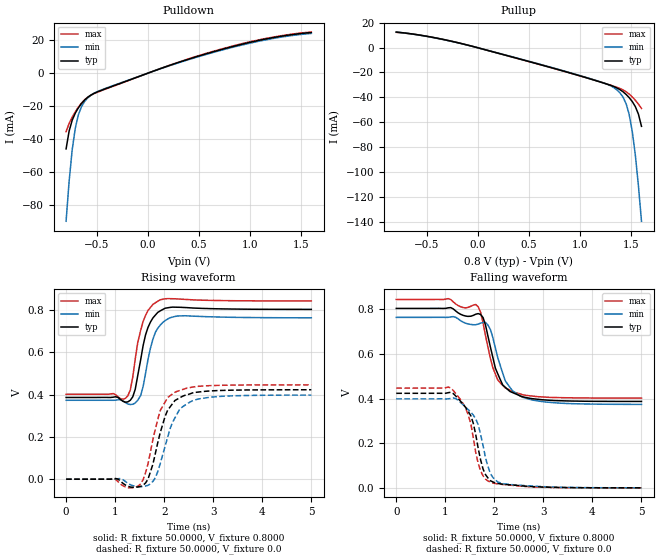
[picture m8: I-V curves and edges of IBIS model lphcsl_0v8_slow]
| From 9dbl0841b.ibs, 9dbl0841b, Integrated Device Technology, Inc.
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|   Model lphcsl_0v8_slow
[Model]  lphcsl_0v8_slow
Model_type Output
Polarity   Non-Inverting
Vmeas =  0.4000V
Cref =   2.0000pF
Rref =   0.0
Vref =   0.4000V
C_comp   1.1000pF   1.0000pF   1.2000pF
[Temperature Range]   27.0000   70.0000   0.0
[Voltage Range]   0.8000V   0.7600V   0.8400V
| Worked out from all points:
|   slope of the pulldown table from 0 to 0.12 V, typ, clamps not added: 44.4 ohm
|   slope of the pullup table from 0 to 0.12 V, typ, clamps not added: 45.4 ohm
|   rising waveform, R_fixture 50.0000, V_fixture 0.8000: 20-80 % time 229ps typ, 225ps min, 222ps max; typ from 0.387 V to 0.804 V
|   rising waveform, R_fixture 50.0000, V_fixture 0.0: 20-80 % time 326ps typ, 359ps min, 314ps max; typ from 0 V to 0.424 V
|   falling waveform, R_fixture 50.0000, V_fixture 0.8000: 20-80 % time 322ps typ, 361ps min, 304ps max; typ from 0.804 V to 0.387 V
|   falling waveform, R_fixture 50.0000, V_fixture 0.0: 20-80 % time 292ps typ, 304ps min, 288ps max; typ from 0.424 V to 0 V
[Pulldown]
|Voltage   I(typ)   I(min)   I(max)
-800mV    -45.83mA   -89.64mA   -35.38mA
-770mV    -34.96mA   -65.18mA   -30.39mA
-740mV    -28.44mA   -46.28mA   -26.61mA
-710mV    -24.18mA   -33.3mA    -23.37mA
-680mV    -20.99mA   -25.25mA   -20.55mA
-650mV    -18.42mA   -20.38mA   -18.13mA
-560mV    -13.36mA   -13.48mA   -13.42mA
-440mV    -10.03mA   -9.766mA   -10.23mA
40mV      915.1uA    880.5uA    940.4uA
610mV     12.43mA    12.04mA    12.7mA
1.15V     20.66mA    20.14mA    20.96mA
1.6V      24.6mA     24.08mA    24.91mA
[Pullup]
|Voltage   I(typ)   I(min)   I(max)
-800mV    12.48mA    12.51mA    12.27mA
-380mV    7.219mA    7.086mA    7.269mA
130mV     -3.031mA   -2.951mA   -3.076mA
1.09V     -24.95mA   -24.74mA   -24.99mA
1.36V     -32.46mA   -34.01mA   -31.91mA
1.42V     -35.56mA   -39.89mA   -34.04mA
1.45V     -37.69mA   -45.23mA   -35.52mA
1.48V     -40.26mA   -53.91mA   -37.39mA
1.51V     -43.39mA   -67.45mA   -39.67mA
1.54V     -47.46mA   -86.58mA   -42.36mA
1.57V     -53.47mA   -111mA     -45.42mA
1.6V      -63.26mA   -139.6mA   -48.89mA
[Ramp]
| variable   typ   min   max
dV/dt_r  0.2541/0.3264n   0.2390/0.3591n   0.2680/0.3137n
dV/dt_f  0.2501/0.3223n   0.2340/0.3607n   0.2651/0.3043n
R_load = 50.0000
[Rising Waveform]
R_fixture= 50.0000
V_fixture= 0.8000
V_fixture_min= 0.7600
V_fixture_max= 0.8400
|time   V(typ)   V(min)   V(max)
0s        387mV      373.7mV    402.1mV
1.21ns    364.7mV    362.8mV    382.7mV
1.31ns    373.9mV    353.4mV    423.1mV
1.36ns    390.4mV    354.9mV    484.2mV
1.52ns    564.4mV    395.7mV    704.5mV
1.67ns    718.5mV    566.8mV    799.1mV
1.77ns    763.4mV    662.4mV    827.3mV
1.92ns    797mV      729.3mV    849.6mV
2.27ns    814.1mV    772.6mV    853.4mV
5ns       804mV      764mV      844mV
[Rising Waveform]
R_fixture= 50.0000
V_fixture= 0.0
V_fixture_min= 0.0
V_fixture_max= 0.0
|time   V(typ)   V(min)   V(max)
0s        0V         0V         0V
1.11ns    -9.201mV   2.827mV    -23.21mV
1.46ns    -36.84mV   -35.36mV   -33.31mV
1.62ns    -17.87mV   -32.01mV   30.65mV
1.82ns    121.8mV    6.681mV    236.7mV
2.02ns    298.1mV    157.4mV    365.9mV
2.27ns    379.2mV    311.9mV    416.5mV
2.53ns    404.3mV    365.9mV    434.2mV
2.93ns    417.6mV    388mV      443mV
5ns       423.5mV    398.4mV    446.7mV
[Falling Waveform]
R_fixture= 50.0000
V_fixture= 0.8000
V_fixture_min= 0.7600
V_fixture_max= 0.8400
|time   V(typ)   V(min)   V(max)
0s        803.9mV    763.8mV    843.9mV
1.16ns    802mV      767.3mV    833.7mV
1.62ns    777.8mV    730.8mV    821.4mV
1.77ns    762.7mV    740.6mV    738.4mV
1.87ns    679mV      729.1mV    629.6mV
2.07ns    510.5mV    582.3mV    483mV
2.22ns    451mV      480.6mV    448.3mV
2.42ns    422.2mV    426.8mV    427.2mV
3.03ns    393.7mV    384.8mV    406.6mV
5ns       387.1mV    373.8mV    402.1mV
[Falling Waveform]
R_fixture= 50.0000
V_fixture= 0.0
V_fixture_min= 0.0
V_fixture_max= 0.0
|time   V(typ)   V(min)   V(max)
0s        423.5mV    398.6mV    446.8mV
1.16ns    422.7mV    402.7mV    436.8mV
1.46ns    344.8mV    351.8mV    331.4mV
1.52ns    323.1mV    339.8mV    287.9mV
1.62ns    239mV      308.8mV    158.6mV
1.67ns    177.4mV    283.1mV    110.4mV
1.77ns    83.93mV    188.7mV    53.6mV
1.92ns    31.74mV    64.24mV    25.1mV
2.22ns    15.19mV    16.92mV    14.08mV
5ns       28.05uV    81.29uV    11.52uV
